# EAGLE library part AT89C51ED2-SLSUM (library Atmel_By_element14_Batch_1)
Microcontroller
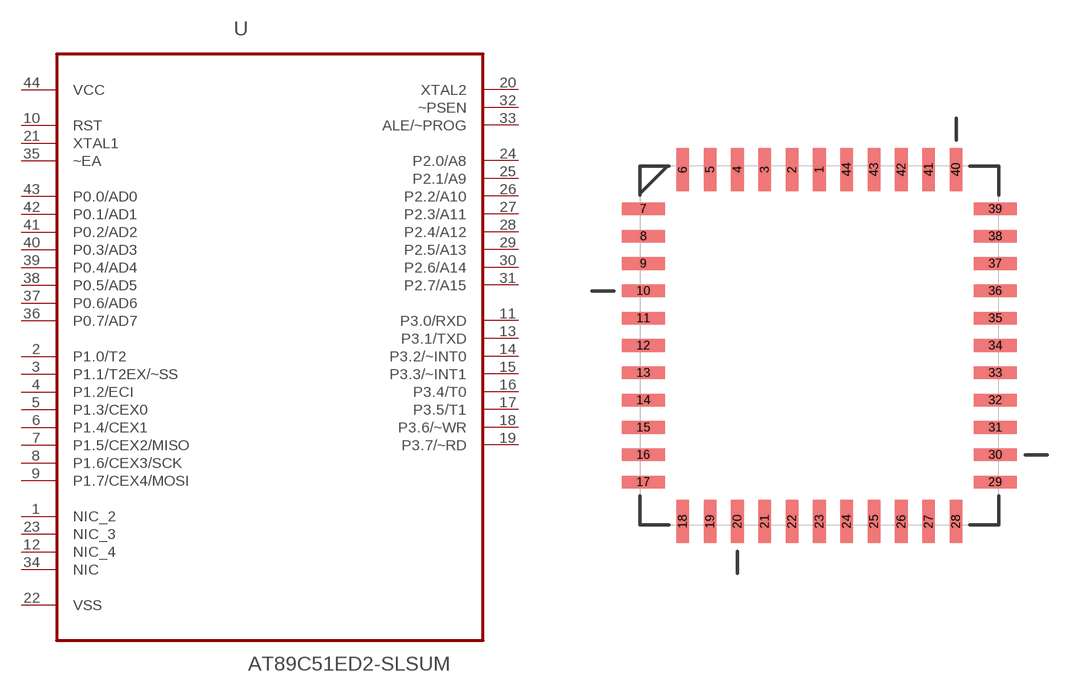
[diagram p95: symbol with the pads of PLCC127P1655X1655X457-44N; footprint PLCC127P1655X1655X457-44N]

Designator prefix U

## AT89C51ED2-SLSUM (DESCRIPTION: Microcontroller; MPN: AT89C51ED2-SLSUM; OC_FARNELL: 1095726; OC_NEWARK: 78K5790; PACKAGE: PLCC-44; SUPPLIER: ATMEL)  [PLCC127P1655X1655X457-44N]
1  NIC_2  nc
2  P1.0/T2
3  P1.1/T2EX/~SS
4  P1.2/ECI
5  P1.3/CEX0
6  P1.4/CEX1
7  P1.5/CEX2/MISO
8  P1.6/CEX3/SCK
9  P1.7/CEX4/MOSI
10  RST  in
11  P3.0/RXD
12  NIC_4  nc
13  P3.1/TXD
14  P3.2/~INT0
15  P3.3/~INT1
16  P3.4/T0
17  P3.5/T1
18  P3.6/~WR
19  P3.7/~RD
20  XTAL2  out
21  XTAL1  in
22  VSS  pwr
23  NIC_3  nc
24  P2.0/A8
25  P2.1/A9
26  P2.2/A10
27  P2.3/A11
28  P2.4/A12
29  P2.5/A13
30  P2.6/A14
31  P2.7/A15
32  ~PSEN  out
33  ALE/~PROG  out
34  NIC  nc
35  ~EA  in
36  P0.7/AD7
37  P0.6/AD6
38  P0.5/AD5
39  P0.4/AD4
40  P0.3/AD3
41  P0.2/AD2
42  P0.1/AD1
43  P0.0/AD0
44  VCC  pwr

## Footprint PLCC127P1655X1655X457-44N (pad centres in mm)
smd 0.584 x 2.007: 1 0,8.179; 2 -1.27,8.179; 3 -2.54,8.179; 4 -3.81,8.179; 5 -5.08,8.179; 6 -6.35,8.179; 18 -6.35,-8.179; 19 -5.08,-8.179; 20 -3.81,-8.179; 21 -2.54,-8.179; 22 -1.27,-8.179; 23 0,-8.179; 24 1.27,-8.179; 25 2.54,-8.179; 26 3.81,-8.179; 27 5.08,-8.179; 28 6.35,-8.179; 40 6.35,8.179; 41 5.08,8.179; 42 3.81,8.179; 43 2.54,8.179; 44 1.27,8.179
smd 2.007 x 0.584: 7 -8.179,6.35; 8 -8.179,5.08; 9 -8.179,3.81; 10 -8.179,2.54; 11 -8.179,1.27; 12 -8.179,0; 13 -8.179,-1.27; 14 -8.179,-2.54; 15 -8.179,-3.81; 16 -8.179,-5.08; 17 -8.179,-6.35; 29 8.179,-6.35; 30 8.179,-5.08; 31 8.179,-3.81; 32 8.179,-2.54; 33 8.179,-1.27; 34 8.179,0; 35 8.179,1.27; 36 8.179,2.54; 37 8.179,3.81; 38 8.179,5.08; 39 8.179,6.35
